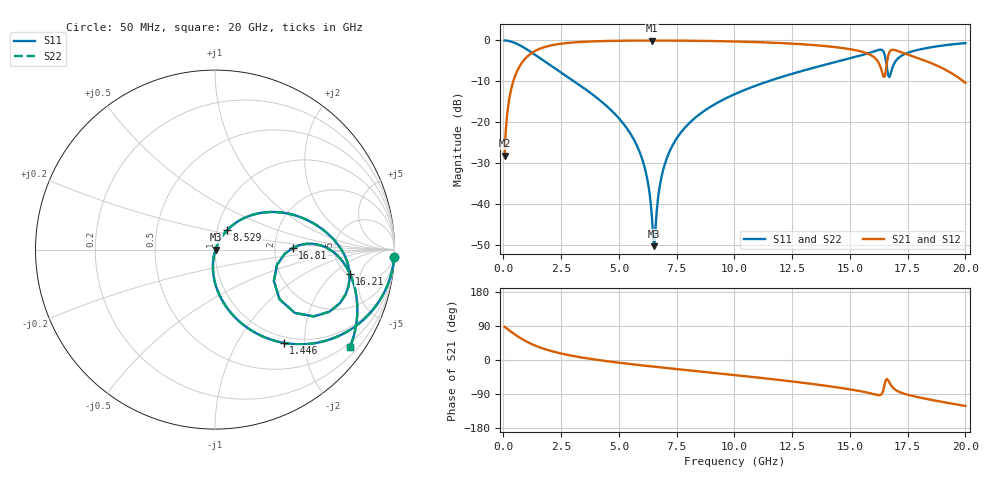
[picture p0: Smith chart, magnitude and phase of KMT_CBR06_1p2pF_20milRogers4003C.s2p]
! Data measured by Modelithics Inc. support@modelithics.com 813-866-6335
! KEMET CBR0603 1.2pF, Pad Width= 0.851mm, Pad Length= 0.64mm, Pad Gap= 0.62mm, 20mil Rogers 4003C substrate Data, January 2022
# hz S ma R 50
! 2 Port Network Data from SP1.SP block
! freq  magS11  angS11  magS21  angS21  magS12  angS12  magS22  angS22
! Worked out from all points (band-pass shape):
!   401 points, 50 MHz to 20 GHz, reference 50 ohm
!   highest |S21| = -0.03 dB at 6.434 GHz (marker M1); lowest = -28.2 dB at 50 MHz (marker M2)
!   |S21| within 3 dB of the highest: 1.238 GHz to 15.67 GHz (14.44 GHz wide, 171 % of centre); 16.7 GHz to 17.29 GHz (592 MHz wide, 3.48 % of centre)
!   lowest |S11| = -50.3 dB at 6.534 GHz (marker M3), VSWR 1.01, Z = 50.3 - j0.0126 ohm
!   |S11| at or under -10 dB: 3.062 GHz to 11.46 GHz (8.397 GHz wide, 116 % of centre)
!   |S22| runs from -50.3 to 0.0 dB; largest |S21 - S12| = 0
!   S11 on the Smith chart (normalised r, x): 50 MHz: 1, -48; 1.446 GHz: 0.90, -1.60; 8.529 GHz: 1.12, +0.25; 16.21 GHz: 5.21, -3.32; 16.81 GHz: 2.53, +0.06; 20 GHz: 0.39, -3.05
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5e7  0.9992 -2.4  0.039 87.6  0.039 87.6  0.9992 -2.4
2.495e8  0.9814 -11.7  0.1914 78.3  0.1914 78.3  0.9814 -11.7
4.98875e8  0.931 -22.7  0.3644 67.2  0.3644 67.2  0.931 -22.7
1.4465e9  0.6454 -53.6  0.7623 36.3  0.7623 36.3  0.6454 -53.6
3.391625e9  0.2724 -83.0  0.9599 6.6  0.9599 6.6  0.2724 -83.0
5.685875e9  0.05848 -99.4  0.9954 -12.1  0.9954 -12.1  0.05848 -99.4
6.184625e9  0.02309 -98.3  0.9967 -15.5  0.9967 -15.5  0.02309 -98.3
6.434e9  0.006573 -80.7  0.9968 -17.1  0.9968 -17.1  0.006573 -80.7
6.53375e9  0.003054 -2.3  0.9968 -17.7  0.9968 -17.7  0.003054 -2.3
6.73325e9  0.01436 58.9  0.9967 -19.0  0.9967 -19.0  0.01436 58.9
6.982625e9  0.03048 63.6  0.9962 -20.6  0.9962 -20.6  0.03048 63.6
7.33175e9  0.05279 63.7  0.9952 -22.9  0.9952 -22.9  0.05279 63.7
8.52875e9  0.1275 58.0  0.988 -30.4  0.988 -30.4  0.1275 58.0
1.0025e10  0.2212 49.1  0.9706 -39.8  0.9706 -39.8  0.2212 49.1
1.336662e10  0.4582 25.8  0.8805 -63.2  0.8805 -63.2  0.4582 25.8
1.531175e10  0.6372 7.7  0.7523 -80.7  0.7523 -80.7  0.6372 7.7
1.62095e10  0.7614 -10.1  0.5534 -92.4  0.5534 -92.4  0.7614 -10.1
1.650875e10  0.6644 -34.1  0.3646 -62.9  0.3646 -62.9  0.6644 -34.1
1.670825e10  0.3559 -13.9  0.7177 -59.5  0.7177 -59.5  0.3559 -13.9
1.6808e10  0.4332 1.2  0.7665 -69.1  0.7665 -69.1  0.4332 1.2
1.78055e10  0.7498 -8.7  0.6285 -96.2  0.6285 -96.2  0.7498 -8.7
2e10  0.9277 -35.8  0.303 -121.1  0.303 -121.1  0.9277 -35.8
